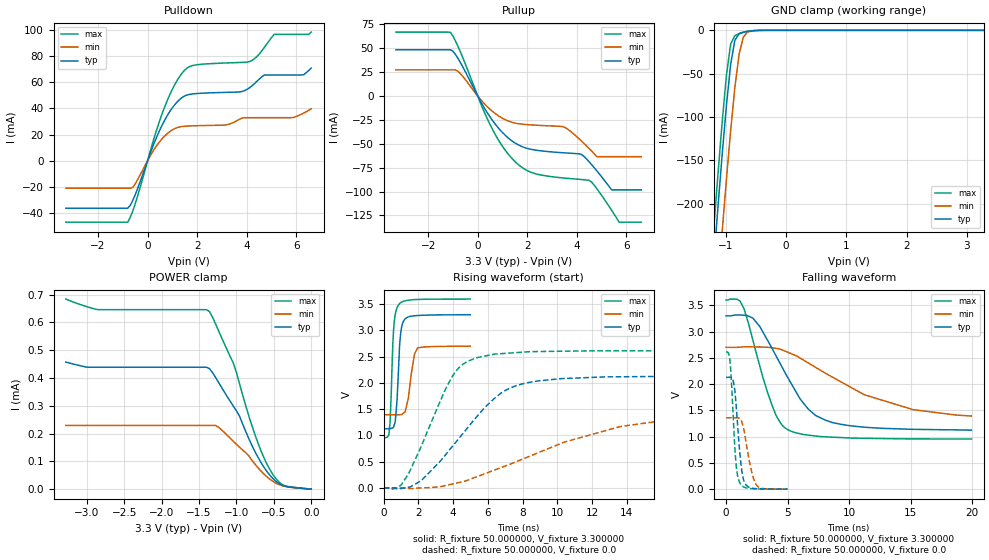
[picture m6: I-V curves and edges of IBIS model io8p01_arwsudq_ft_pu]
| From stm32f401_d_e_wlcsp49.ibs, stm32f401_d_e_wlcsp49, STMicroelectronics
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|   Model io8p01_arwsudq_ft_pu
[Model]  io8p01_arwsudq_ft_pu
Model_type I/O
Polarity   Non-Inverting
Enable   Active-Low
Vinl =   0.990000V
Vinh =   2.310000V
Vmeas =  1.650000V
Cref =   50.000000pF
Rref =   100.000000M
Vref =   0.0V
C_comp   2.905500pF   2.823600pF   2.987900pF
[Temperature Range]   25.000000   0.125000k   -40.000000
[Pullup Reference]   3.300000V   2.700000V   3.600000V
[Pulldown Reference]   0.0V   0.0V   0.0V
[POWER Clamp Reference]   3.300000V   2.700000V   3.600000V
[GND Clamp Reference]   0.0V   0.0V   0.0V
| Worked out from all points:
|   slope of the pulldown table from 0 to 0.495 V, typ, clamps not added: 20.9 ohm
|   slope of the pullup table from 0 to 0.495 V, typ, clamps not added: 22.6 ohm
|   GND clamp passes 1 mA (typ) near -0.62 V on its own axis
|   rising waveform, R_fixture 50.000000, V_fixture 3.300000: 20-80 % time 212ps typ, 338ps min, 188ps max; typ from 1.12 V to 3.3 V
|   rising waveform, R_fixture 50.000000, V_fixture 0.0: 20-80 % time 3.35ns typ, 6.89ns min, 2.1ns max; typ from 0.001 V to 2.13 V
|   falling waveform, R_fixture 50.000000, V_fixture 3.300000: 20-80 % time 3.26ns typ, 6.81ns min, 2.01ns max; typ from 3.3 V to 1.12 V
|   falling waveform, R_fixture 50.000000, V_fixture 0.0: 20-80 % time 461ps typ, 654ps min, 373ps max; typ from 2.13 V to 0.001 V
[Pulldown]
|Voltage   I(typ)   I(min)   I(max)
-3.3V     -36.39mA   -21.07mA   -47.09mA
-800mV    -36.39mA   -21.07mA   -47.09mA
-600mV    -30.5mA    -20.54mA   -38.69mA
700mV     31.4mA     19.11mA    41.71mA
1.2V      45.15mA    25.37mA    61.75mA
1.6V      50.35mA    26.5mA     71.06mA
3.1V      52.28mA    27.26mA    74.75mA
4.1V      55.65mA    32.92mA    75.79mA
4.7V      65.56mA    32.92mA    86.49mA
5.1V      65.56mA    32.92mA    96.69mA
6.3V      65.85mA    36.49mA    96.69mA
6.6V      70.9mA     39.7mA     98.44mA
[Pullup]
|Voltage   I(typ)   I(min)   I(max)
-3.3V     48.41mA    27.39mA    66.93mA
-1.1V     48.41mA    27.39mA    66.7mA
-700mV    35.09mA    23.45mA    46.27mA
500mV     -22.06mA   -14mA      -30.02mA
1.5V      -49.1mA    -28.3mA    -68.56mA
2.2V      -56.04mA   -30.32mA   -80.35mA
3.5V      -59.52mA   -32.65mA   -85.91mA
4.5V      -69.08mA   -55.12mA   -88.39mA
4.8V      -78.23mA   -63.5mA    -96.87mA
5.4V      -98.3mA    -63.5mA    -119.6mA
5.7V      -98.3mA    -63.5mA    -132.1mA
6.6V      -98.3mA    -63.5mA    -132.1mA
[GND_clamp]
|Voltage   I(typ)   I(min)   I(max)
-3.3V     -2.319A    -2.397A    -2.292A
-1.2V     -266mA     -356.2mA   -228.4mA
-1.13V    -203.2mA   -293mA     -165.3mA
-1.06V    -142.7mA   -231.3mA   -105.2mA
-990mV    -86.51mA   -171.7mA   -51.78mA
-920mV    -39.3mA    -115.7mA   -15.93mA
-850mV    -11.37mA   -65.76mA   -6.097mA
-780mV    -3.83mA    -27.55mA   -3.88mA
-710mV    -2.09mA    -7.747mA   -2.382mA
-640mV    -1.147mA   -2.129mA   -1.22mA
-570mV    -523.9uA   -800uA     -476.9uA
3.28V     0A         0A         0A
[POWER_clamp]
|Voltage   I(typ)   I(min)   I(max)
-3.28V    457.2uA    229.4uA    683.8uA
-2.84V    438.5uA    229.4uA    645.6uA
-1.36V    433.5uA    229.4uA    638.5uA
-1.24V    384.6uA    223.2uA    570.8uA
-1.04V    298.3uA    171.8uA    452.6uA
-960mV    263.4uA    151.4uA    380.6uA
-760mV    139.5uA    92.81uA    202.3uA
-640mV    82.23uA    56.4uA     118uA
-560mV    52.51uA    37.37uA    73.96uA
-440mV    21.63uA    17.4uA     27.8uA
-360mV    11.48uA    10.27uA    13.1uA
0V        0A         0A         0A
[Ramp]
| variable   typ   min   max
dV/dt_r  1.27741/3.35096n   0.79905/6.89895n   1.56693/2.10274n
dV/dt_f  1.30152/3.25476n   0.73968/6.77388n   1.58713/2.00710n
R_load = 50.000000
[Rising Waveform]
R_fixture= 50.000000
V_fixture= 3.300000
V_fixture_min= 2.700000
V_fixture_max= 3.600000
|time   V(typ)   V(min)   V(max)
0s        1.125V     1.393V     955.6mV
300.3ps   1.127V     1.393V     1.014V
370.4ps   1.129V     1.393V     1.256V
570.6ps   1.16V      1.393V     3.004V
670.7ps   1.272V     1.393V     3.311V
830.8ps   2.087V     1.393V     3.473V
981ps     2.949V     1.396V     3.53V
1.241ns   3.223V     1.457V     3.565V
1.962ns   3.285V     2.67V      3.591V
4.985ns   3.3V       2.7V       3.599V
[Rising Waveform]
R_fixture= 50.000000
V_fixture= 0.0
V_fixture_min= 0.0
V_fixture_max= 0.0
|time   V(typ)   V(min)   V(max)
0s        1.449mV    1.249mV    1.825mV
1.001ns   -11.65mV   65.27uV    52.52mV
2.162ns   137.1mV    220.9uV    792mV
3.924ns   777.7mV    71.59mV    2.107V
4.565ns   1.038V     119.6mV    2.357V
5.325ns   1.344V     207.8mV    2.478V
7.007ns   1.859V     418.2mV    2.564V
8.889ns   2.039V     669mV      2.599V
13.61ns   2.118V     1.168V     2.612V
19.94ns   2.129V     1.36V      2.612V
[Falling Waveform]
R_fixture= 50.000000
V_fixture= 3.300000
V_fixture_min= 2.700000
V_fixture_max= 3.600000
|time   V(typ)   V(min)   V(max)
0s        3.3V       2.7V       3.599V
920.9ps   3.315V     2.7V       3.611V
1.441ns   3.312V     2.71V      3.44V
2.202ns   3.25V      2.71V      2.817V
3.764ns   2.668V     2.69V      1.582V
5.005ns   2.128V     2.608V     1.135V
6.647ns   1.533V     2.408V     1.031V
8.609ns   1.271V     2.137V     991.7mV
15.18ns   1.14V      1.516V     957.8mV
19.94ns   1.125V     1.393V     955.6mV
[Falling Waveform]
R_fixture= 50.000000
V_fixture= 0.0
V_fixture_min= 0.0
V_fixture_max= 0.0
|time   V(typ)   V(min)   V(max)
0s        2.129V     1.36V      2.612V
300.3ps   2.131V     1.359V     2.482V
620.6ps   2.024V     1.359V     1.198V
820.8ps   1.596V     1.361V     457.3mV
1.091ns   767.8mV    1.353V     135.4mV
1.291ns   335.1mV    1.281V     65.89mV
1.481ns   141.9mV    1.093V     38.75mV
2.142ns   19.53mV    270mV      9.623mV
2.452ns   11.6mV     86.06mV    7.128mV
4.985ns   1.449mV    1.249mV    1.825mV
